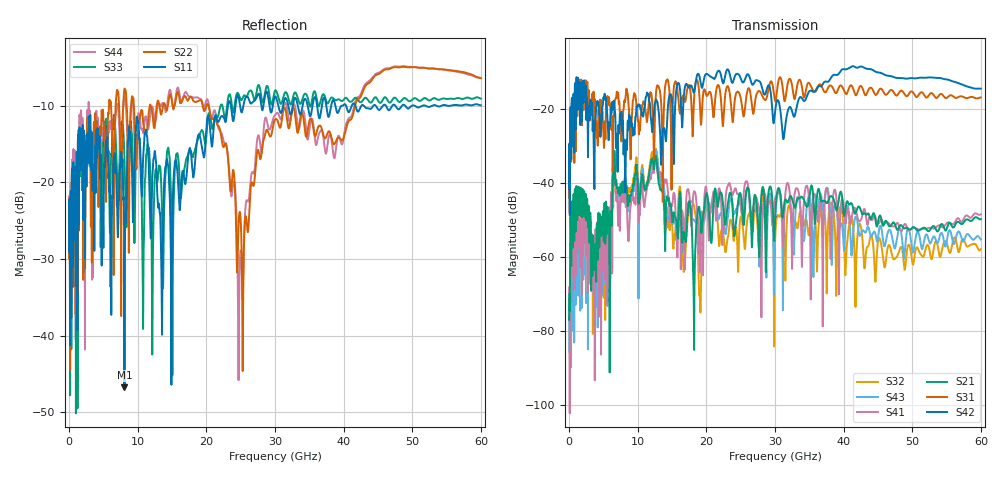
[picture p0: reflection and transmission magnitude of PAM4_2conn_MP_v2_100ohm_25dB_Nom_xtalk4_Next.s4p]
! Info: Touchstone file created by Circ.  Input file=FAB50GbE_2conn_Midplane_Examax_Topo2_v2_100ohm_25dB_Nom.circ
# Hz S RI R 50
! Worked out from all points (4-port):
!   6000 points, 10 MHz to 60 GHz, reference 50 ohm
!   strongest paths, dB at 10 MHz, 15.01 GHz, 30.01 GHz, 45.01 GHz, 60 GHz:
!     S42: -41.7, -18.2, -20.8, -10.2, -14.6
!     S31: -43.9, -25.5, -17.9, -15.5, -16.9
!     S21: -76.2, -49.7, -50.4, -50.6, -49.8
!     S41: -68.2, -46.2, -44.3, -51.0, -48.5
!     S43: -71.3, -49.4, -50.4, -54.9, -55.3
!     S32: -75.2, -51.4, -56.3, -55.9, -57.9
!   lowest |S11| = -46.8 dB at 8.07 GHz (marker M1), VSWR 1.01, Z = 49.6 + j0.134 ohm
!   |S11| at or under -10 dB: start of sweep to 23.14 GHz; 42.96 GHz to 44.31 GHz (1.349 GHz wide, 3.09 % of centre); 44.7 GHz to 45.71 GHz (1.015 GHz wide, 2.25 % of centre)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
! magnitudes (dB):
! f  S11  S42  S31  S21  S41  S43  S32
! 10 MHz  -29.1  -41.7  -43.9  -76.2  -68.2  -71.3  -75.2
! 1.09 GHz  -16.3  -11.5  -12.7  -41.1  -48.1  -54.3  -49.1
! 8.07 GHz  -46.8  -29.2  -17.8  -39.5  -45.3  -45.1  -41.5
! 18.2 GHz  -18.9  -15.6  -17.8  -78.7  -42.4  -50.0  -46.1
! 19.04 GHz  -14.0  -11.6  -17.9  -47.7  -63.1  -58.9  -70.5
! 24.87 GHz  -9.7  -11.1  -16.1  -42.8  -44.4  -45.2  -51.0
! 60 GHz  -9.9  -14.6  -16.9  -49.8  -48.5  -55.3  -57.9
